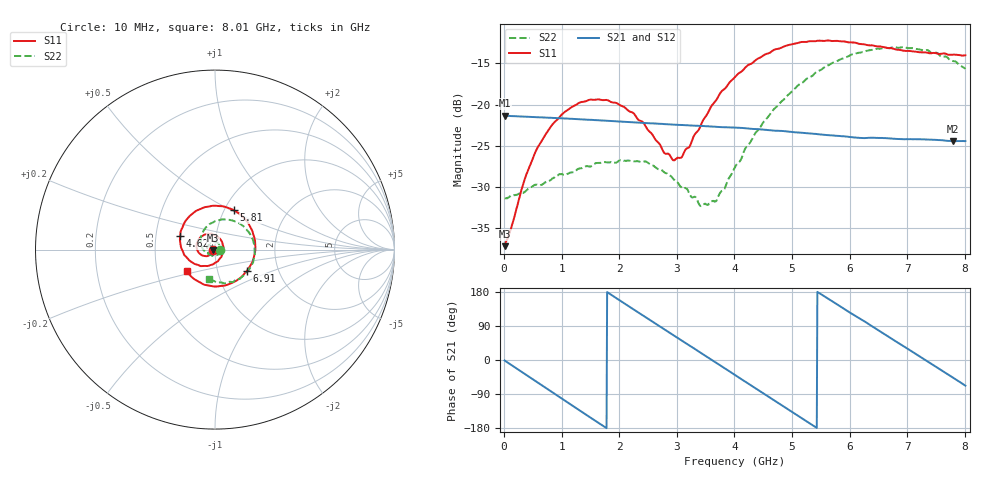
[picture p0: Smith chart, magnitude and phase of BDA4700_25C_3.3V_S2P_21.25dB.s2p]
!Agilent Technologies,E5071B,MY42404982,A.09.10
!Date: Mon Oct 20 18:11:59 2025
!Data & Calibration Information:
!Freq	S11:SOLT2(ON)	S21:SOLT2(ON)	S12:SOLT2(ON)	S22:SOLT2(ON)
# Hz S RI R 50
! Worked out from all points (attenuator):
!   801 points, 10 MHz to 8.01 GHz, reference 50 ohm
!   highest |S21| = -21.33 dB at 10 MHz (marker M1); lowest = -24.4 dB at 7.8 GHz (marker M2)
!   lowest |S11| = -37.2 dB at 10 MHz (marker M3), VSWR 1.03, Z = 48.6 - j0.134 ohm
!   |S11| at or under -10 dB: start of sweep to end of sweep
!   |S22| runs from -32.3 to -13.0 dB; largest |S21 - S12| = 0.00098
!   S11 on the Smith chart (normalised r, x): 10 MHz: 0.97, -0.00; 4.62 GHz: 0.67, +0.11; 5.81 GHz: 1.11, +0.52; 6.91 GHz: 1.38, -0.34; 8.01 GHz: 0.71, -0.18
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1e7  -0.0137 -0.00137  0.0858 -0.00185  0.0858 -0.00192  0.0269 -0.000818
3.7e8  -0.0246 -0.0263  0.0666 -0.0521  0.0665 -0.0521  0.0223 -0.0196
5.8e8  -0.0413 -0.0357  0.0427 -0.0722  0.0428 -0.0721  0.0144 -0.0292
1e9  -0.0832 -0.0245  -0.0168 -0.0808  -0.0167 -0.0809  -0.0148 -0.0349
1.35e9  -0.1031 0.0127  -0.0594 -0.0556  -0.0593 -0.0556  -0.0369 -0.0181
2.07e9  -0.0433 0.0871  -0.0691 0.0378  -0.0691 0.0378  -0.0305 0.0341
2.68e9  0.0386 0.0441  -0.0014 0.0765  -0.00146 0.0764  0.014 0.038
2.93e9  0.0461 0.00198  0.0301 0.0694  0.0301 0.0692  0.0258 0.0246
3.06e9  0.0424 -0.0214  0.0447 0.0606  0.0441 0.0608  0.0285 0.0145
3.43e9  -0.0036 -0.0768  0.0708 0.0223  0.0708 0.0223  0.0199 -0.0139
3.69e9  -0.0567 -0.0909  0.0726 -0.0102  0.0726 -0.0104  0.000892 -0.0261
4.01e9  -0.1292 -0.0702  0.0559 -0.0462  0.056 -0.0461  -0.0321 -0.0264
4.62e9  -0.1928 0.0758  -0.0119 -0.0688  -0.0118 -0.0688  -0.079 0.0377
4.96e9  -0.1549 0.1709  -0.0468 -0.0499  -0.0467 -0.0502  -0.0694 0.094
5.35e9  -0.0486 0.2377  -0.0659 -0.00994  -0.0658 -0.0103  -0.0159 0.1485
5.81e9  0.1056 0.2191  -0.0523 0.0378  -0.0521 0.0378  0.087 0.1642
6.25e9  0.2075 0.105  -0.0137 0.0611  -0.0127 0.0613  0.1816 0.105
6.68e9  0.2155 -0.047  0.0305 0.0544  0.0306 0.0544  0.2207 -0.00198
6.91e9  0.1772 -0.119  0.048 0.0386  0.0482 0.0384  0.2133 -0.0671
7.34e9  0.049 -0.2008  0.0613 -0.00295  0.0614 -0.00294  0.1414 -0.1608
7.8e9  -0.1079 -0.1698  0.0407 -0.044  0.0407 -0.0441  0.0174 -0.183
8.01e9  -0.1584 -0.1212  0.0227 -0.0556  0.0229 -0.0555  -0.0325 -0.1619
